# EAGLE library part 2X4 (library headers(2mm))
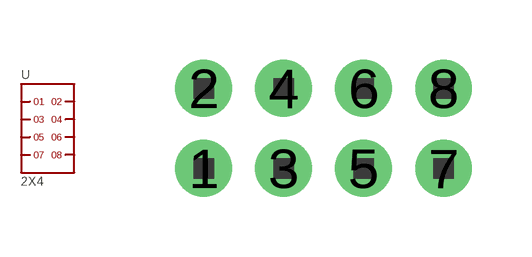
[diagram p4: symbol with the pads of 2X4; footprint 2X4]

Designator prefix -

## 2X4  [2X4]
1  1
2  2
3  3
4  4
5  5
6  6
7  7
8  8

## Footprint 2X4 (pad centres in mm)
drill 0.8 pad 1.422: 1 -3,-1; 2 -3,1; 3 -1,-1; 4 -1,1; 5 1,-1; 6 1,1; 7 3,-1; 8 3,1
